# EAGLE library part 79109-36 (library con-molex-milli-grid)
RECEPTACAL
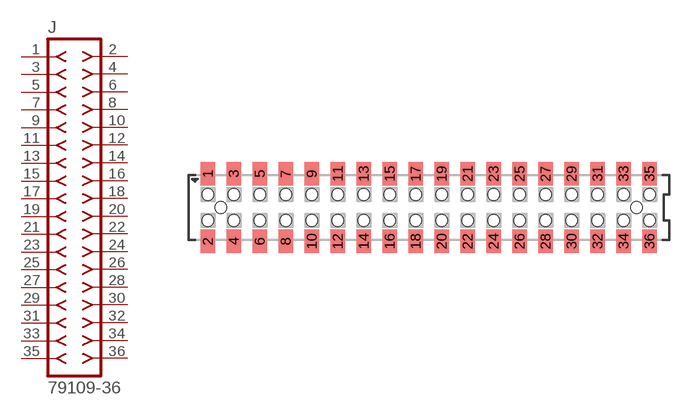
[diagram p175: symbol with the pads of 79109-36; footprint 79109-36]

Designator prefix J

## 79109-36  [79109-36]
1  1  pas
2  2  pas
3  3  pas
4  4  pas
5  5  pas
6  6  pas
7  7  pas
8  8  pas
9  9  pas
10  10  pas
11  11  pas
12  12  pas
13  13  pas
14  14  pas
15  15  pas
16  16  pas
17  17  pas
18  18  pas
19  19  pas
20  20  pas
21  21  pas
22  22  pas
23  23  pas
24  24  pas
25  25  pas
26  26  pas
27  27  pas
28  28  pas
29  29  pas
30  30  pas
31  31  pas
32  32  pas
33  33  pas
34  34  pas
35  35  pas
36  36  pas

## Footprint 79109-36 (pad centres in mm)
RECEPTACAL SMD Dual Row, Vertical, Pass-Thru
smd 1.12 x 1.83: 1 -17,2.6; 2 -17,-2.6; 3 -15,2.6; 4 -15,-2.6; 5 -13,2.6; 6 -13,-2.6; 7 -11,2.6; 8 -11,-2.6; 9 -9,2.6; 10 -9,-2.6; 11 -7,2.6; 12 -7,-2.6; 13 -5,2.6; 14 -5,-2.6; 15 -3,2.6; 16 -3,-2.6; 17 -1,2.6; 18 -1,-2.6; 19 1,2.6; 20 1,-2.6; 21 3,2.6; 22 3,-2.6; 23 5,2.6; 24 5,-2.6; 25 7,2.6; 26 7,-2.6; 27 9,2.6; 28 9,-2.6; 29 11,2.6; 30 11,-2.6; 31 13,2.6; 32 13,-2.6; 33 15,2.6; 34 15,-2.6; 35 17,2.6; 36 17,-2.6
hole 0.914 at -16,0
hole 0.914 at -17,1
hole 0.914 at -17,-1
hole 0.914 at -15,-1
hole 0.914 at -15,1
hole 0.914 at -13,-1
hole 0.914 at -13,1
hole 0.914 at 16,0
hole 0.914 at -11,1
hole 0.914 at -11,-1
hole 0.914 at -9,1
hole 0.914 at -9,-1
hole 0.914 at -7,1
hole 0.914 at -7,-1
hole 0.914 at -5,1
hole 0.914 at -5,-1
hole 0.914 at -3,-1
hole 0.914 at -3,1
hole 0.914 at -1,1
hole 0.914 at -1,-1
hole 0.914 at 1,1
hole 0.914 at 1,-1
hole 0.914 at 3,1
hole 0.914 at 3,-1
hole 0.914 at 5,-1
hole 0.914 at 5,1
hole 0.914 at 7,1
hole 0.914 at 9,1
hole 0.914 at 11,1
hole 0.914 at 7,-1
hole 0.914 at 9,-1
hole 0.914 at 11,-1
hole 0.914 at 13,-1
hole 0.914 at 15,-1
hole 0.914 at 17,-1
hole 0.914 at 13,1
hole 0.914 at 15,1
hole 0.914 at 17,1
